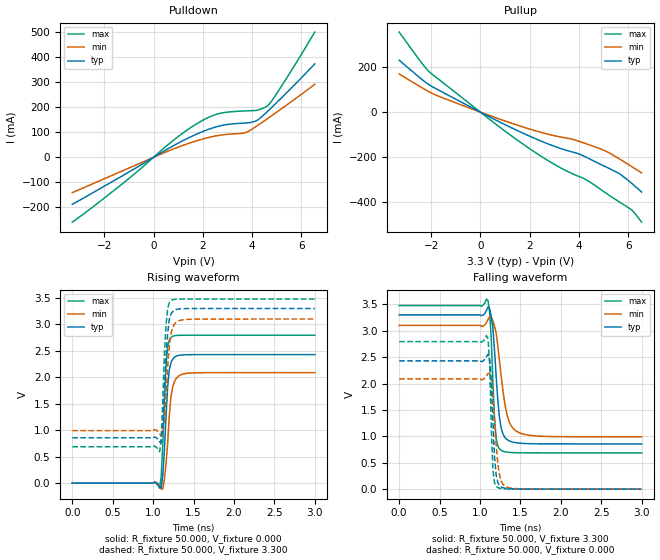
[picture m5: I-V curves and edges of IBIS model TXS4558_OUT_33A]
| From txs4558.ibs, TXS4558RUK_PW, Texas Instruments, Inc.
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[Model]   TXS4558_OUT_33A
Model_type  Output
Vref =   1.65
Rref =   50
Cref =   15p
Vmeas =   1.65
| variable   typ   min   max
C_comp   2.07pF   0.95pF   3.66pF
| C_pullup   1.86pF   0.95pF   3.58pF
| C_pulldown   2.28pF   1.15pF   3.66pF
[Temperature Range]   40   100   -40
| Ambient temperature   25   85   -40
[Voltage range]   3.3   3.15   3.45
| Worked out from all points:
|   slope of the pulldown table from 0 to 0.495 V, typ, clamps not added: 17.1 ohm
|   slope of the pullup table from 0 to 0.495 V, typ, clamps not added: 17.7 ohm
|   falling waveform, R_fixture 50.000, V_fixture 3.300: 20-80 % time 71.3ps typ, 112ps min, 47.9ps max; typ from 3.3 V to 0.857 V
|   rising waveform, R_fixture 50.000, V_fixture 0.000: 20-80 % time 53.9ps typ, 62.9ps min, 46.8ps max; typ from 0 V to 2.43 V
|   rising waveform, R_fixture 50.000, V_fixture 3.300: 20-80 % time 50.7ps typ, 59ps min, 46ps max; typ from 0.856 V to 3.3 V
|   falling waveform, R_fixture 50.000, V_fixture 0.000: 20-80 % time 45.1ps typ, 62.5ps min, 33ps max; typ from 2.43 V to 0 V
[Pulldown]
| TXS4558_OUT_33A
|   Voltage   I(typ)   I(min)   I(max)
-3.3V     -187.5mA   -140.8mA   -258.7mA
-1.32V    -76.94mA   -56.46mA   -110.1mA
858mV     48.95mA    35.1mA     71.68mA
1.798V    94.46mA    67.31mA    136.2mA
2.244V    111.9mA    79.22mA    159.6mA
2.64V     123.9mA    87.11mA    173.7mA
3.729V    136.6mA    98.46mA    185mA
4.175V    145.7mA    123.3mA    187.4mA
4.62V     181.8mA    153.5mA    204.3mA
4.769V    195.8mA    163.7mA    220.3mA
5.066V    224.2mA    184.3mA    263.2mA
6.551V    372.4mA    291.1mA    499.3mA
[Pullup]
|   Voltage   I(typ)   I(min)   I(max)
-3.3V     231.2mA    169.9mA    356.3mA
-2.458V   153mA      114.1mA    229.5mA
-2.112V   124mA      92.4mA     183.1mA
165mV     -9.385mA   -6.686mA   -14.25mA
1.353V    -74.2mA    -52.54mA   -112.8mA
2.442V    -127.7mA   -89.33mA   -194.7mA
3.284V    -162.6mA   -111.1mA   -249.4mA
4.026V    -187mA     -130.6mA   -287.4mA
4.917V    -234.2mA   -164.8mA   -346.4mA
5.61V     -271.3mA   -205.5mA   -397.3mA
6.105V    -313mA     -239.4mA   -431.9mA
6.551V    -355.8mA   -270.4mA   -489.8mA
[Ramp]
R_load = 50
|   typ   min   max
dV/dt_r   1.45698/5.38894e-11   1.19356/6.28278e-11   1.749/4.67885e-11
dV/dt_f   1.46594/7.13553e-11   1.20456/1.11643e-10   1.74761/4.79328e-11
[Falling Waveform]
R_fixture = 50.000
V_fixture = 3.300
V_fixture_min = 3.000
V_fixture_max = 3.600
C_fixture = 0.000
|  time   V(typ)   V(min)   V(max)
0s        3.3V       3.101V     3.478V
1.1ns     3.452V     3.214V     3.57V
1.14ns    3.264V     3.249V     2.844V
1.16ns    3.053V     3.184V     2.026V
1.18ns    2.626V     3.086V     1.336V
1.2ns     2.142V     2.959V     963.7mV
1.26ns    1.172V     2.174V     737.3mV
1.34ns    933.9mV    1.378V     700.1mV
1.48ns    873mV      1.073V     689.4mV
3ns       856.8mV    992.1mV    687.2mV
[Rising Waveform]
R_fixture = 50.000
V_fixture = 0.000
V_fixture_min = 0.000
V_fixture_max = 0.000
C_fixture = 0.000
|  time   V(typ)   V(min)   V(max)
0s        3.495nV    4.358uV    -5.434uV
1.08ns    -81.28mV   -42.84mV   -93.57mV
1.1ns     -97.84mV   -114.5mV   119.5mV
1.12ns    155.8mV    -105.4mV   743.4mV
1.16ns    1.26V      367.2mV    2.22V
1.18ns    1.819V     748.9mV    2.578V
1.2ns     2.138V     1.264V     2.704V
1.24ns    2.337V     1.803V     2.773V
1.42ns    2.426V     2.075V     2.794V
3ns       2.428V     2.088V     2.794V
[Rising Waveform]
R_fixture = 50.000
V_fixture = 3.300
V_fixture_min = 3.000
V_fixture_max = 3.600
C_fixture = 0.000
|  time   V(typ)   V(min)   V(max)
0s        856.5mV    992.1mV    687.2mV
1.08ns    776.5mV    945.1mV    592.3mV
1.1ns     773.2mV    890.2mV    819.4mV
1.12ns    1.07V      932.2mV    1.557V
1.14ns    1.705V     1.18V      2.45V
1.16ns    2.385V     1.658V     2.986V
1.18ns    2.826V     2.206V     3.299V
1.22ns    3.19V      2.815V     3.445V
1.4ns     3.298V     3.092V     3.478V
3ns       3.3V       3.101V     3.478V
[Falling Waveform]
R_fixture = 50.000
V_fixture = 0.000
V_fixture_min = 0.000
V_fixture_max = 0.000
C_fixture = 0.000
|  time   V(typ)   V(min)   V(max)
0s        2.429V     2.088V     2.794V
1.08ns    2.509V     2.144V     2.908V
1.1ns     2.555V     2.189V     2.846V
1.12ns    2.458V     2.201V     2.367V
1.16ns    1.265V     1.781V     364.6mV
1.18ns    609mV      1.308V     121.5mV
1.22ns    131mV      494.2mV    31.52mV
1.28ns    30.42mV    101.5mV    9.06mV
1.38ns    7.914mV    21.04mV    2.279mV
3ns       245.9uV    4.358uV    -5.434uV
